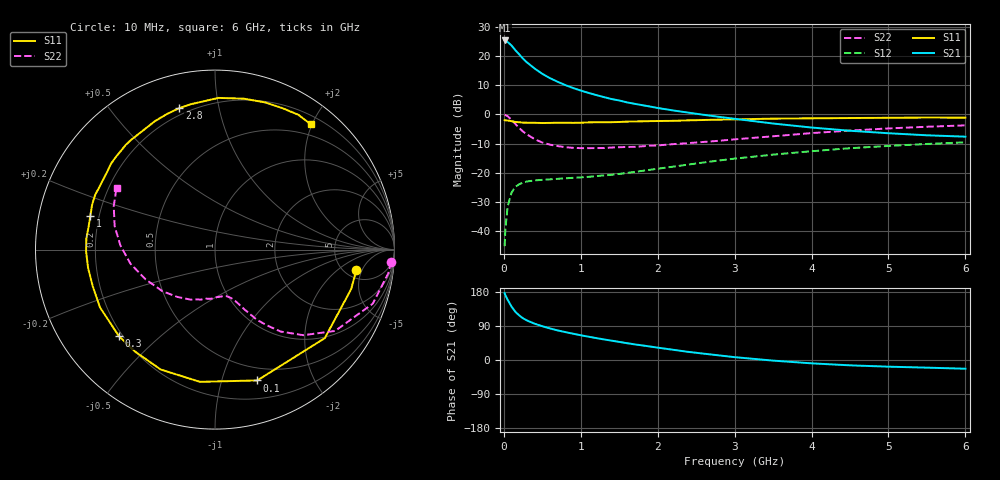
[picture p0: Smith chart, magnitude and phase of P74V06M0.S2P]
! SIEMENS Small Signal Semiconductors
! BFP196
! Si NPN RF Bipolar Junction Transistor in SOT143
! VCE = 4 V  IC = 6 mA
! Common Emitter S-Parameters:  May  1996
# GHz  S  MA  R  50
!  f  S11  S21  S12  S22
! GHz  MAG  ANG  MAG  ANG  MAG  ANG  MAG  ANG
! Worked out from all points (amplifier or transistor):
!   36 points, 10 MHz to 6 GHz, reference 50 ohm
!   highest |S21| = 25.4 dB at 10 MHz (marker M1)
!   |S21| within 3 dB of that: start of sweep to 139.2 MHz
!   unconditionally stable (mu >= 1): 1.075 GHz to 3.135 GHz
!   at 250 MHz: K = 0.29, MSG = 21.2 dB, |S12| = -23.4 dB
!   at 1.4 GHz: K = 1.17, MAG = 10.5 dB, |S12| = -20.7 dB
!   at 6 GHz: K = 0.99, MSG = 1.0 dB, |S12| = -9.6 dB
!   S11 on the Smith chart (normalised r, x): 10 MHz: 6.33, -3.92; 100 MHz: 0.37, -1.31; 300 MHz: 0.19, -0.37; 1 GHz: 0.17, +0.13; 2.8 GHz: 0.16, +0.77; 6 GHz: 0.32, +1.99
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0.01  0.7958 -8.2  18.52 176.5  0.0055 85.3  0.9836 -4.0
0.02  0.79 -16.2  18.04 170.9  0.0107 81.4  0.9749 -7.7
0.05  0.7859 -38.9  17.4 158.6  0.0266 70.9  0.9293 -18.9
0.1  0.766 -72.1  15.16 140.9  0.0455 56.1  0.8083 -34.1
0.15  0.7416 -96.5  12.6 127.1  0.0573 45.4  0.6852 -44.1
0.2  0.7334 -114.4  10.69 117.6  0.0634 38.4  0.5852 -51.3
0.25  0.722 -128.2  9.008 109.9  0.0677 33.8  0.5067 -55.9
0.3  0.7202 -138.1  7.794 104.4  0.0707 30.8  0.4545 -59.2
0.4  0.7172 -153.4  6.117 95.8  0.0738 26.9  0.3761 -63.5
0.5  0.7111 -163.4  4.958 89.1  0.0754 25.2  0.3291 -66.6
0.6  0.7145 -171.8  4.176 83.3  0.077 25.0  0.3025 -69.0
0.8  0.7194 175.1  3.177 73.6  0.0801 25.7  0.2744 -73.9
1  0.7196 164.7  2.562 65.3  0.0832 28.3  0.2638 -79.1
1.1  0.729 159.9  2.336 61.5  0.085 29.5  0.2637 -81.9
1.3  0.7327 151.4  1.98 54.3  0.09 32.1  0.2648 -87.7
1.6  0.7512 140.6  1.608 44.4  0.0991 35.9  0.2763 -96.8
2.2  0.7751 121.2  1.169 27.0  0.1269 40.3  0.309 -115.4
2.8  0.8127 104.2  0.906 12.1  0.1622 39.0  0.353 -135.5
3.5  0.8454 88.7  0.697 -1.6  0.2041 33.4  0.4213 -156.9
4.5  0.8663 71.2  0.524 -14.1  0.2631 22.4  0.5279 177.4
5.5  0.8831 58.2  0.438 -20.2  0.3112 10.3  0.6138 156.8
6  0.8787 52.5  0.415 -23.0  0.3318 3.7  0.6481 147.8
